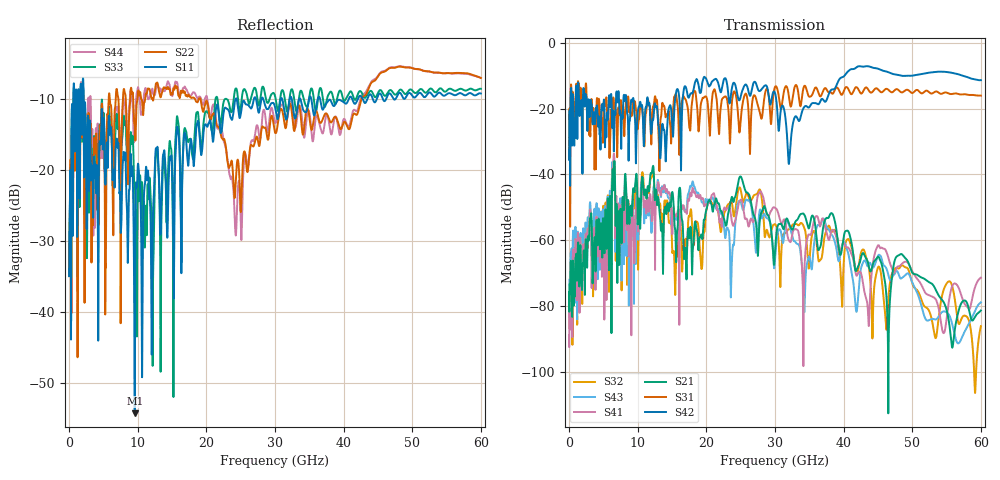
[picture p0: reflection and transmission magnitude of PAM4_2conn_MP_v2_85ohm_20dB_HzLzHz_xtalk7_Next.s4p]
! Info: Touchstone file created by Circ.  Input file=FAB50GbE_2conn_Midplane_Examax_Topo2_v2_85ohm_20dB_HzLzHz.circ
# Hz S RI R 50
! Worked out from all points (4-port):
!   6000 points, 10 MHz to 60 GHz, reference 50 ohm
!   strongest paths, dB at 10 MHz, 15.01 GHz, 30.01 GHz, 45.01 GHz, 60 GHz:
!     S42: -35.5, -24.0, -15.3, -7.9, -11.4
!     S31: -35.4, -22.8, -13.4, -14.2, -16.0
!     S21: -75.7, -45.4, -63.2, -65.0, -81.3
!     S41: -88.7, -57.3, -50.1, -61.5, -71.3
!     S43: -77.4, -53.2, -65.6, -64.7, -78.8
!     S32: -81.9, -62.3, -55.1, -68.2, -86.0
!   lowest |S11| = -54.2 dB at 9.57 GHz (marker M1), VSWR 1.00, Z = 49.8 + j0.0928 ohm
!   |S11| at or under -10 dB: 2.123 GHz to 24.29 GHz (22.17 GHz wide, 168 % of centre); 28.28 GHz to 30.86 GHz (2.575 GHz wide, 8.71 % of centre); 36.56 GHz to 40.76 GHz (4.196 GHz wide, 10.9 % of centre)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
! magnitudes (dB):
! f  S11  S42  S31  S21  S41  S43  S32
! 10 MHz  -34.9  -35.5  -35.4  -75.7  -88.7  -77.4  -81.9
! 870 MHz  -15.3  -25.2  -24.5  -72.5  -65.3  -59.4  -64.1
! 6.4 GHz  -20.3  -20.8  -17.4  -40.5  -41.6  -39.9  -39.2
! 9.57 GHz  -54.2  -22.2  -17.9  -44.5  -62.7  -52.6  -49.0
! 15.54 GHz  -17.3  -15.8  -15.5  -60.9  -52.3  -53.4  -69.7
! 27.69 GHz  -11.9  -14.7  -20.4  -56.6  -45.7  -52.0  -44.6
! 60 GHz  -9.3  -11.4  -16.0  -81.3  -71.3  -78.8  -86.0
